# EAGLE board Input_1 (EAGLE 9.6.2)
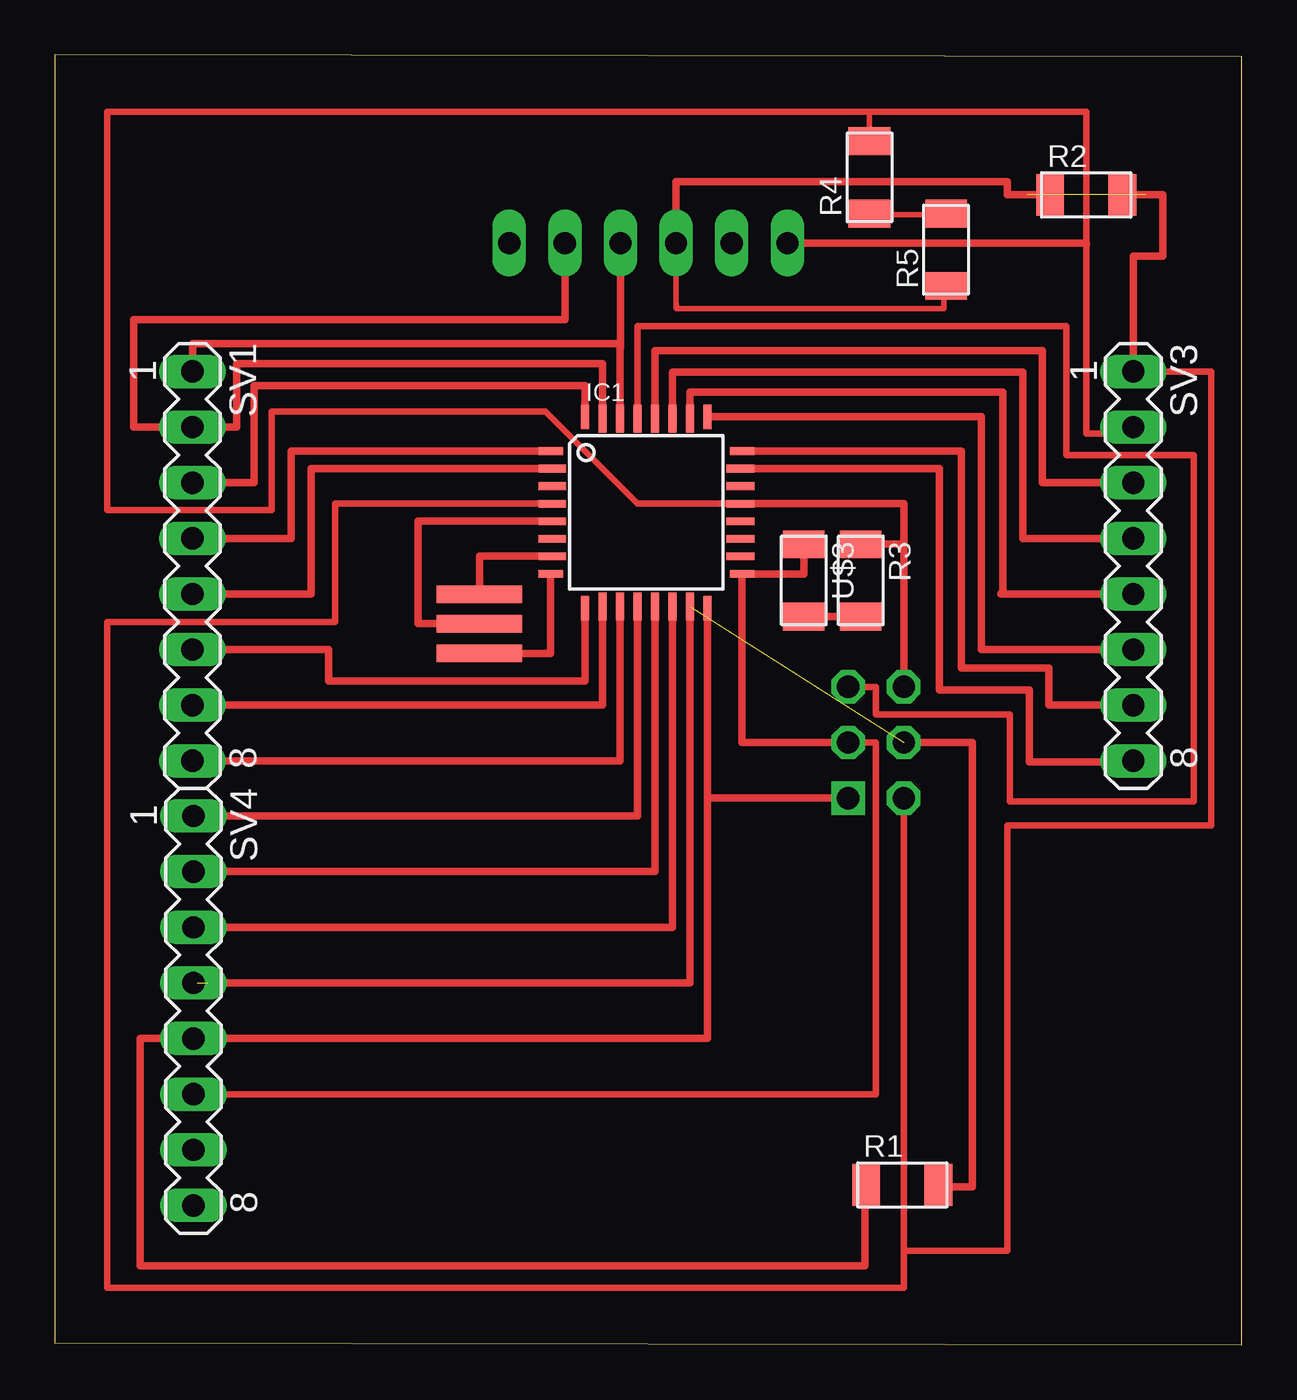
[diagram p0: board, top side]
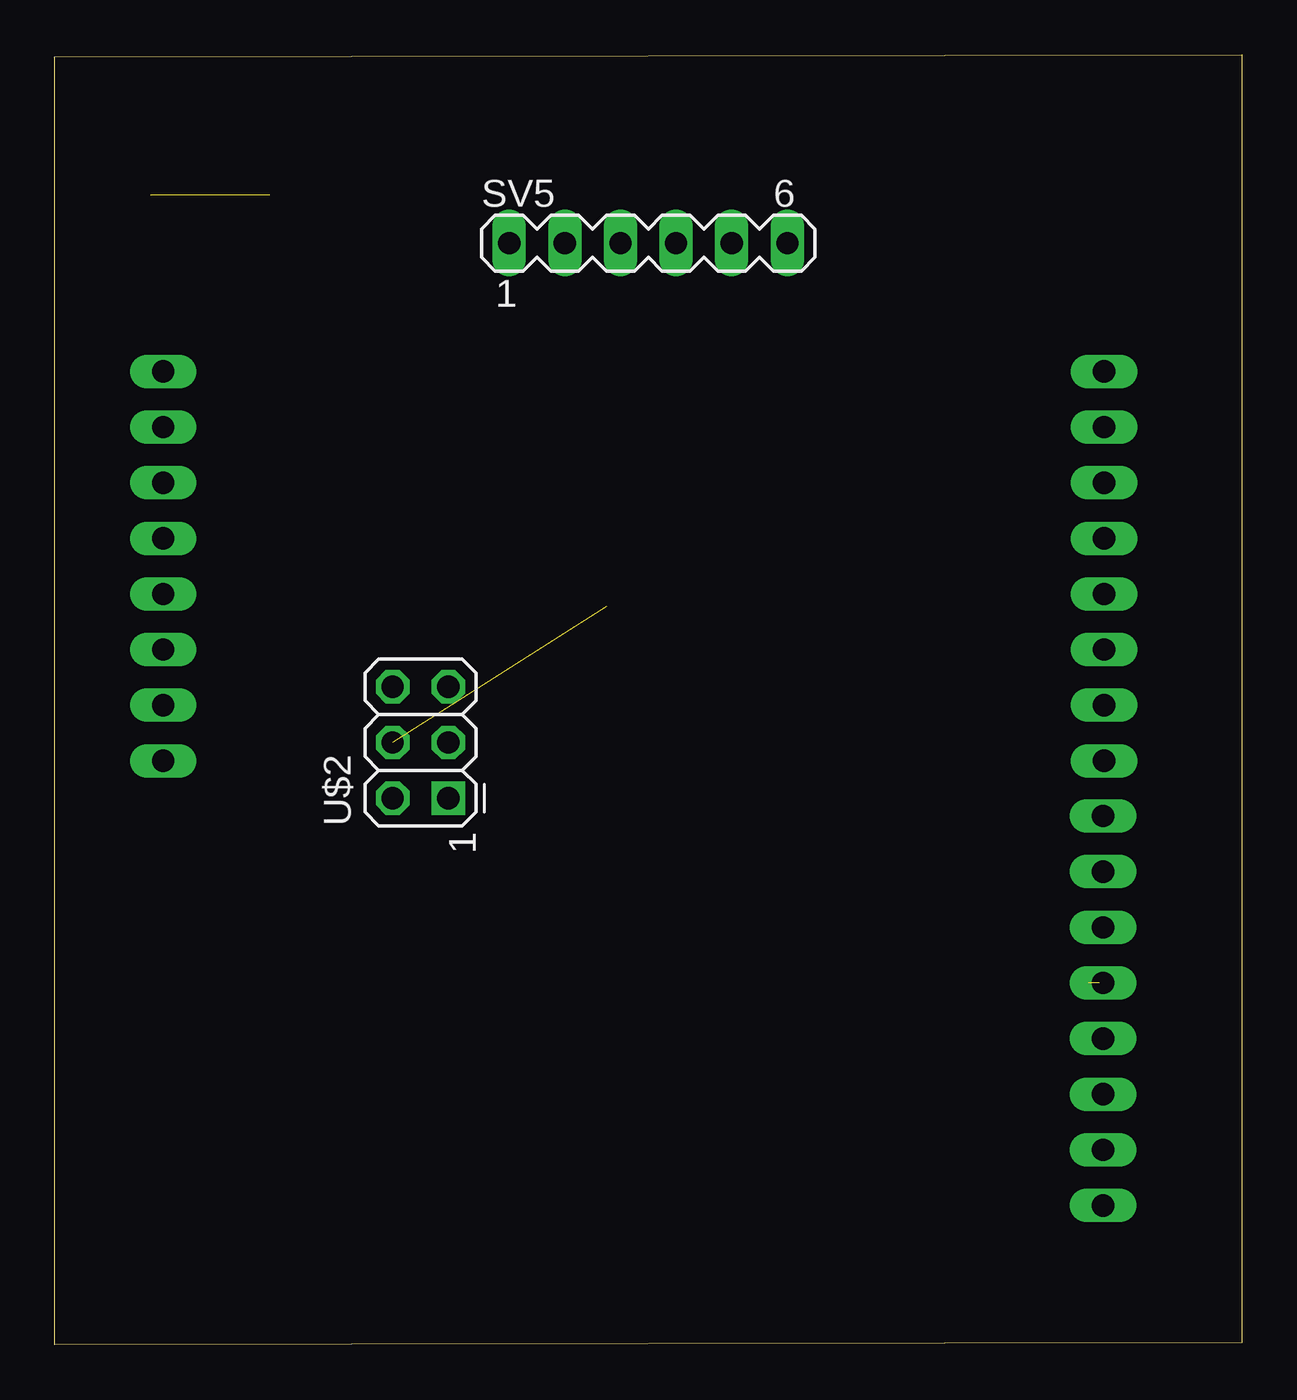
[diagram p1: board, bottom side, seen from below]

Size 54.2 x 58.9 mm. Coordinates in mm from the lower left corner, seen from the top.
Outline: 0,0.1 54.2,0 54.2,58.8 0,58.9 0,0.1
Copper layers (1*16): Top 0.035mm / dielectric 1.5mm / Bottom 0.035mm
Design rules "default *": minimum track width 10mil, minimum drill 0.35mm, track to track 10mil, track to pad 10mil, pad to pad 10mil, via to via 10mil, smd to smd 10mil, copper to edge 40mil, drill to drill 6mil, minimum pad ring 10mil, minimum via ring 8mil, stop-mask expansion 4mil, vias tented up to drill 0mil, thermal gap 10mil

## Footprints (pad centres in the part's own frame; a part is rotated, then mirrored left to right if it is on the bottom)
TQFP32-08THIN = smd 1.118 x 0.356: 1 -4.369,2.8; 8 -4.369,-2.8; 17 4.369,-2.8; 24 4.369,2.8 | smd 1.27 x 0.356: 2 -4.293,2; 3 -4.293,1.2; 4 -4.293,0.4; 5 -4.293,-0.4; 6 -4.293,-1.2; 7 -4.293,-2; 18 4.293,-2; 19 4.293,-1.2; 20 4.293,-0.4; 21 4.293,0.4; 22 4.293,1.2; 23 4.293,2 | smd 0.356 x 1.118: 9 -2.8,-4.369; 16 2.8,-4.369; 25 2.8,4.369; 32 -2.8,4.369 | smd 0.356 x 1.27: 10 -2,-4.293; 14 1.2,-4.293; 15 2,-4.293; 26 2,4.293; 27 1.2,4.293; 31 -2,4.293 | smd 0.35 x 1.27: 11 -1.2,-4.293; 12 -0.4,-4.293; 13 0.4,-4.293; 28 0.4,4.293; 29 -0.4,4.293; 30 -1.2,4.293
R1206FAB = smd 1.27 x 1.905: 1 -1.651,0; 2 1.651,0
MA08-1 = drill 1.016 long: 1 -8.89,0; 2 -6.35,0; 3 -3.81,0; 4 -1.27,0; 5 1.27,0; 6 3.81,0; 7 6.35,0; 8 8.89,0
MA06-1 = drill 1.016 long: 1 -6.35,0; 2 -3.81,0; 3 -1.27,0; 4 1.27,0; 5 3.81,0; 6 6.35,0
EFOBM = smd 0.8 x 3.9: 1 -1.35,0; 2 0,0; 3 1.35,0
2X03 = drill 1.016 square: 1 -2.54,-1.27 | drill 1.016 octagon: 2 -2.54,1.27; 3 0,-1.27; 4 0,1.27; 5 2.54,-1.27; 6 2.54,1.27
LED1206FAB = smd 1.27 x 1.905: 1 -1.651,0; 2 1.651,0

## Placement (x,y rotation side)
IC1  ATMEGA88-THIN  [TQFP32-08THIN]  27.01,38 0 top
R1  [R1206FAB]  38.7,7.3 0 top
R2  [R1206FAB]  47.1,52.5 0 top
R3  [R1206FAB]  36.8,34.9 270 top
R4  [R1206FAB]  37.2,53.3 90 top
R5  [R1206FAB]  40.7,50 90 top
SV1  [MA08-1]  6.29,35.55 270 top
SV3  [MA08-1]  49.25,35.55 270 top
SV4  [MA08-1]  6.33,15.25 270 top
SV5  [MA06-1]  27.1,50.3 0 bottom
U$1  RESONATOR  [EFOBM]  19.39,32.92 270 top
U$2  AVRISP  [2X03]  37.5,27.5 90 bottom
U$3  LEDFAB1206  [LED1206FAB]  34.2,34.9 270 top

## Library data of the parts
IC1 R1-R5 U$1-U$3 = fab
SV1 SV3-SV5 = con-lstb; OC_FARNELL: unknown; OC_NEWARK: unknown

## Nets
AVCC: IC1.18
GND: IC1.3
N$1: IC1.7 U$1.1
N$2: IC1.8 U$1.3
N$3: IC1.21 R3.1 SV3.2 SV5.1 U$2.6
N$4: IC1.16 SV4.5 U$2.1
N$5: IC1.15 SV4.4 U$2.4
N$6: IC1.17 SV4.6 U$2.3 U$3.1
N$7: IC1.29 U$2.5
N$8: IC1.4 SV3.1 SV5.3 U$2.2
N$9: IC1.30 SV1.1 SV5.4
N$10: IC1.31 SV1.2 SV5.5
N$11: IC1.32 SV1.3
N$12: IC1.1 SV1.4
N$13: IC1.2 SV1.5
N$14: IC1.9 SV1.6
N$15: IC1.10 SV1.7
N$16: IC1.11 SV1.8
N$17: IC1.12 SV4.1
N$18: IC1.13 SV4.2
N$19: IC1.14 SV4.3
N$23: IC1.5 U$1.2
N$24: IC1.23 SV3.8
N$25: IC1.24 SV3.7
N$26: IC1.25 SV3.6
N$27: IC1.26 SV3.5
N$28: IC1.27 SV3.4
N$29: IC1.28 SV3.3
N$30: R3.2 U$3.2
VCC: IC1.6

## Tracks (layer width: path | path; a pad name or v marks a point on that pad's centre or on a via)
N$1
  Top 0.35: IC1.7 19.39,36 U$1.1
N$2
  Top 0.35: U$1.3 22.64,31.57 IC1.8
N$3
  Top 0.254: 37.2,56.3 37.2,55.4
  Top 0.3: IC1.21 26.6,38.4 22.4,42.6 9.9,42.6 9.9,38.1 2.4,38.1 2.4,56.3 37.2,56.3 47.1,56.3 47.1,50.3 | 47.1,50.2 47.1,41.6 49.25,41.6 SV3.2
  Top 0.35: IC1.21 38.77,38.4 38.77,36.55 | 38.77,36.55 U$2.6 | R3.1 38.77,36.55 | SV5.1 47.1,50.3 47.1,50.2
N$4
  Top 0.35: IC1.16 29.81,24.96 | 29.81,24.96 U$2.1 | 29.81,24.96 29.81,13.98 SV4.5 3.9,13.98 3.9,3.6 37,3.6 37,7.2
N$5  (2 unrouted)
  Top 0.35: SV4.4 6.5,16.52 | 7,16.52 29.01,16.52 IC1.15 | U$2.4 41.9,27.5 41.9,7.2 41.5,7.2 41.41,7.2 40.3,7.2
N$6
  Top 0.3: SV4.6 37.5,11.44 37.5,27.5 U$2.3
  Top 0.35: U$2.3 31.38,27.5 IC1.17 34.2,35.2 U$3.1
N$7
  Top 0.3: U$2.5 37.5,30.04 37.5,28.77 43.6,28.77 43.6,24.8 52,24.8 52,40.63 46.2,40.63 46.2,46.5 26.61,46.5 IC1.29
N$8  (1 unrouted)
  Top 0.254: SV5.3 28.37,47.33
  Top 0.3: IC1.4 12.8,38.4 12.8,33 2.4,33 2.4,2.6 38.77,2.6 38.77,4.3 | 38.77,4.3 U$2.2 | SV3.1 52.8,44.44 52.8,23.7 43.5,23.7 43.5,4.3 38.77,4.3
  Top 0.35: SV5.3 28.37,53.1 43.5,53.1 43.5,52.5 44.38,52.5 | SV3.1 49.25,49.7 50.6,49.7 50.6,52.5 49.81,52.5
N$9
  Top 0.35: IC1.30 25.81,45.5 | 25.81,45.5 25.81,45.7 6.29,45.7 SV1.1 | SV5.4 25.83,45.5 25.81,45.5
N$10
  Top 0.35: IC1.31 25.01,44.8 8.3,44.8 8.3,41.9 SV1.2 3.6,41.9 3.6,46.8 23.3,46.8 SV5.5
N$11
  Top 0.35: SV1.3 9.1,39.36 9.1,43.8 24.21,43.8 IC1.32
N$12
  Top 0.35: IC1.1 10.8,40.8 10.8,36.8 6.29,36.8 SV1.4
N$13
  Top 0.35: SV1.5 11.7,34.28 11.7,40 IC1.2
N$14
  Top 0.35: SV1.6 12.5,31.74 12.5,30.3 24.21,30.3 IC1.9
N$15
  Top 0.35: SV1.7 25.01,29.2 IC1.10
N$16
  Top 0.35: SV1.8 25.81,26.66 IC1.11
N$17
  Top 0.35: IC1.12 26.61,24.14 SV4.1
N$18
  Top 0.35: IC1.13 27.41,21.6 SV4.2
N$19
  Top 0.35: IC1.14 28.21,19.06 SV4.3
N$20
  Top 0.254: 40.6,51.6 37.5,51.6
N$21
  Top 0.254: 40.6,47.4 40.6,48.3
N$22
  Top 0.35: 6.4,16.6 6.4,16.5
N$23
  Top 0.35: U$1.2 16.6,32.92 16.6,37.6 IC1.5
N$24
  Top 0.35: IC1.23 40.4,40 40.4,29.9 44.5,29.9 44.5,26.6 49.25,26.6 SV3.8
N$25
  Top 0.35: IC1.24 41.4,40.8 41.4,30.9 45.4,30.9 45.4,29.2 SV3.7
N$26
  Top 0.35: IC1.25 42.3,42.37 42.3,31.74 SV3.6
N$27
  Top 0.35: IC1.26 29.01,43.5 43.3,43.5 43.3,34.3 43.2,34.3 43.2,34.28 SV3.5
N$28
  Top 0.35: IC1.27 28.21,44.4 44.2,44.4 44.2,36.8 49.25,36.8 SV3.4
N$29
  Top 0.35: IC1.28 27.41,45.4 45.1,45.4 45.1,39.36 SV3.3
N$30
  Top 0.35: U$3.2 R3.2
N$31
  Top 0.35: 49.8,52.5 49,52.5
N$32
  Top 0.35: 44.4,52.5 45.1,52.5
N$33
  Top 0.254: 40.6,47.3 28.4,47.3 28.4,47.5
